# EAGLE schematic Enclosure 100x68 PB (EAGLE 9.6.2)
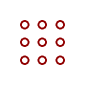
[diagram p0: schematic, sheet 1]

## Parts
U$1  PROTO-34X22  [PROTO-34X22]

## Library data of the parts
U$1 = digitalconcepts:PROTO-34X22: 34 x 22 Prototyping board to fit an 100 x 68 enclosure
